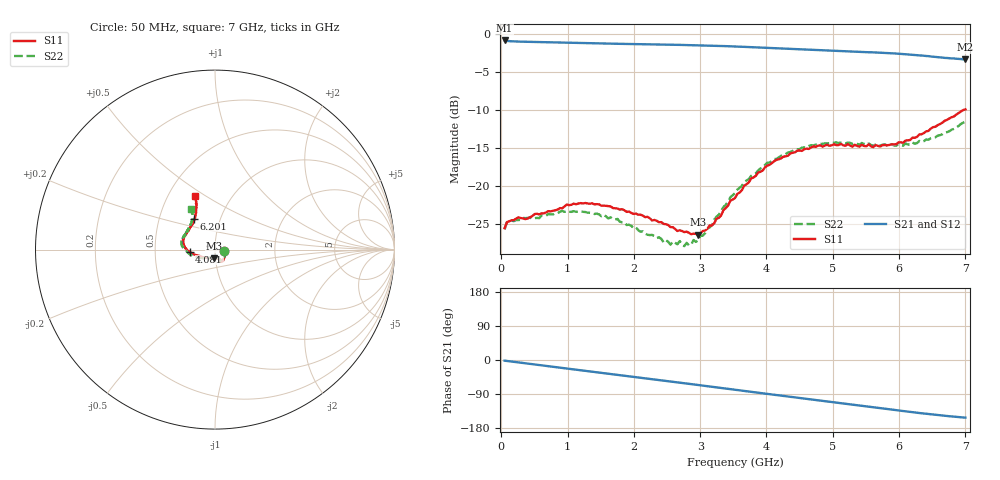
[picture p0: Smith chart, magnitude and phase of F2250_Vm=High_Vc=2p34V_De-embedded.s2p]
! Integrated Device Technology
! Corporate Headquarters
! 6024 Silver Creek Valley Road
! San Jose, CA 95138  USA
! Phone:  1-408-284-8200
! Toll Free:  1-800-223-1366
! Webpage:  http://www.idt.com/
! Timing and RF Division
! 515 Groton Road, Suite 102
! Westford, MA 01886-6024
! Device:  F2250
! Description: Voltage Variable RF Attenuator
! Frequency:  50.0 -  6000.00 MHz
! Package:  3x3 mm Thin QFN Plastic Package: 16 pin
! Ports:  2 RF, 3 DC
!  Pin  1  = GND
!  Pin  2  = NC
!  Pin  3  = RF1  = Port 1
!  Pin  4  = NC
!  Pin  5  = GND
!  Pin  6  = GND
!  Pin  7  = GND
!  Pin  8  = GND
!  Pin  9  = NC
!  Pin 10  = RF2  = Port 2
!  Pin 11  = NC
!  Pin 12  = GND
!  Pin 13  = GND
!  Pin 14  = VCNTRL
!  Pin 15  = VDD
!  Pin 16  = VMODE
! Vcntrl:  2.340 Volts
! Vmode:  +3.300 Volts
! Vdd:  +3.30  Volts
! Current:  1.314 mA
! Data:  The device was measured on a the F2250 evaluation board which has
!  individual transmission lines to the RF pins.  Data was collected
!  using a calibrated network analyzer.  The evaluation board was
!  de-embedded using a TRL calibration technique.
!  The reference plane is the edge of the package pin.
! Misc:  SN 10
!  Action Tracker AT0258
! Date Measured:  2014-11-26
! Date:  2015-10-15  MJV
! Note:
!  Integrated Device Technology supplies this data as a sample of measured
!  data at the package pin for this product.  Your particular data for this
!  product may vary.
!  Data was taken at 25 degrees C.
!  Integrated Device Technology reserves the right to change this data at anytime.
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# GHz S dB R 50
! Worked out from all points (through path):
!   201 points, 50 MHz to 7 GHz, reference 50 ohm
!   highest |S21| = -0.90 dB at 50 MHz (marker M1); lowest = -3.4 dB at 7 GHz (marker M2)
!   group delay of S21, straight-line fit = 61.2 ps
!   lowest |S11| = -26.4 dB at 2.969 GHz (marker M3), VSWR 1.10, Z = 49.2 - j4.7 ohm
!   |S11| at or under -10 dB: start of sweep to 6.975 GHz
!   |S22| runs from -27.9 to -11.5 dB; largest |S21 - S12| = 0.0019
!   S11 on the Smith chart (normalised r, x): 50 MHz: 1.11, -0.02; 4.081 GHz: 0.75, -0.02; 6.201 GHz: 0.75, +0.27; 7 GHz: 0.68, +0.45
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0.05  -25.50 -10.5  -0.90 -1.8  -0.90 -1.8  -25.67 -10.7
0.1195  -24.60 -10.1  -0.99 -3.2  -0.99 -3.2  -24.55 -8.8
0.57125  -23.70 -31.0  -1.11 -13.3  -1.11 -13.3  -24.20 -31.2
0.91875  -22.90 -49.6  -1.18 -21.0  -1.18 -21.1  -23.24 -50.7
1.2315  -22.27 -57.4  -1.25 -27.9  -1.25 -27.9  -23.36 -61.3
1.75275  -22.93 -64.3  -1.34 -39.1  -1.34 -39.1  -24.29 -67.7
2.37825  -24.72 -64.1  -1.43 -52.8  -1.43 -52.8  -26.71 -67.1
2.552  -25.37 -68.9  -1.45 -56.7  -1.45 -56.7  -27.67 -73.4
2.691  -25.79 -76.9  -1.48 -59.8  -1.48 -59.8  -27.20 -81.1
2.7605  -26.02 -79.1  -1.49 -61.3  -1.49 -61.3  -27.86 -85.6
2.969  -26.38 -96.9  -1.53 -66.0  -1.53 -66.0  -27.11 -104.9
3.1775  -25.15 -119.9  -1.58 -70.7  -1.58 -70.7  -25.12 -126.6
3.525  -21.55 -152.1  -1.69 -78.5  -1.69 -78.6  -20.91 -148.6
3.76825  -18.99 -164.3  -1.78 -84.0  -1.78 -84.1  -18.65 -159.6
4.081  -16.98 -175.3  -1.91 -91.0  -1.91 -91.0  -16.69 -171.4
4.4285  -15.56 176.3  -2.04 -98.6  -2.04 -98.7  -15.17 178.7
4.7065  -14.79 169.3  -2.14 -104.8  -2.14 -104.8  -14.67 173.0
5.054  -14.63 161.2  -2.27 -112.5  -2.26 -112.5  -14.27 166.0
5.85325  -14.60 135.3  -2.57 -130.0  -2.57 -130.1  -14.67 147.2
6.20075  -13.65 123.7  -2.78 -137.7  -2.78 -137.8  -14.25 138.2
6.54825  -12.21 115.7  -3.05 -144.7  -3.05 -144.9  -13.59 126.9
7  -9.93 110.9  -3.38 -152.1  -3.39 -152.2  -11.55 120.7
